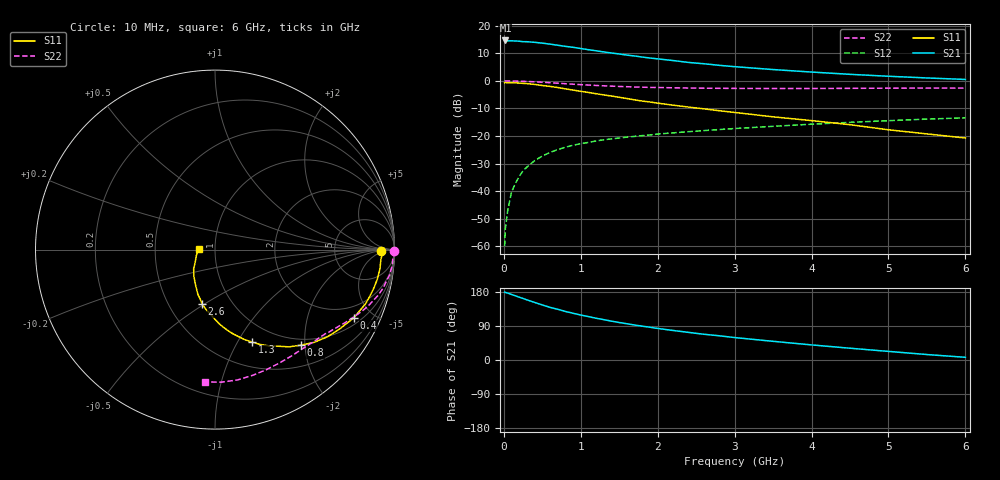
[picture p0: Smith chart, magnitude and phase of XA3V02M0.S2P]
! SIEMENS Discrete & RF Semiconductors
! BFY180
! Si NPN RF Bipolar Junction Transistor in MICRO-X
! VCE = 3 V  IC = 2 mA
! Common Emitter S-Parameters:  May  1997
# GHz  S  MA  R  50
!  f  S11  S21  S12  S22
! GHz  MAG  ANG  MAG  ANG  MAG  ANG  MAG  ANG
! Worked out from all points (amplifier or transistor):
!   36 points, 10 MHz to 6 GHz, reference 50 ohm
!   highest |S21| = 14.7 dB at 20 MHz (marker M1)
!   |S21| within 3 dB of that: start of sweep to 1.018 GHz
!   unconditionally stable (mu >= 1): 2.747 GHz to end of sweep
!   at 250 MHz: K = 0.12, MSG = 23.4 dB, |S12| = -32.6 dB
!   at 1.4 GHz: K = 0.69, MSG = 15.6 dB, |S12| = -21.1 dB
!   at 6 GHz: K = 1.07, MAG = 5.3 dB, |S12| = -13.4 dB
!   S11 on the Smith chart (normalised r, x): 10 MHz: 26, -2; 400 MHz: 1.31, -3.88; 800 MHz: 0.88, -1.91; 1.3 GHz: 0.77, -1.15; 2.6 GHz: 0.73, -0.49; 6 GHz: 0.83, +0.01
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0.01  0.9257 -0.4  5.296 179.1  0.001 82.6  0.9951 -0.3
0.02  0.9326 -1.3  5.411 178.3  0.0021 91.3  0.9958 -0.6
0.05  0.9261 -3.4  5.315 176.5  0.0044 84.4  0.9955 -1.6
0.1  0.9251 -6.7  5.321 173.0  0.0096 87.5  0.9913 -3.4
0.2  0.9109 -13.5  5.246 165.7  0.0184 81.5  0.9866 -6.6
0.25  0.9009 -16.8  5.145 162.4  0.0234 80.5  0.9827 -8.4
0.4  0.8616 -26.2  5.004 151.9  0.0356 73.7  0.9615 -12.8
0.5  0.8242 -32.3  4.837 145.3  0.0432 69.9  0.9443 -15.6
0.6  0.7935 -37.7  4.643 138.9  0.0502 67.1  0.9245 -18.1
0.8  0.7155 -48.1  4.225 128.1  0.0625 61.2  0.888 -22.7
0.9  0.6812 -52.7  4.066 123.3  0.0679 58.6  0.8699 -24.7
1.1  0.6165 -60.6  3.673 114.5  0.0764 55.1  0.839 -28.3
1.3  0.5553 -68.1  3.348 106.5  0.0853 51.5  0.8131 -31.5
1.5  0.5028 -74.8  3.071 98.9  0.0918 48.8  0.7918 -34.5
1.7  0.4517 -81.6  2.829 92.2  0.0983 47.1  0.7733 -37.3
2  0.394 -89.2  2.505 83.3  0.1084 44.5  0.7576 -41.3
2.2  0.3621 -93.9  2.339 77.9  0.1138 42.6  0.7487 -44.0
2.6  0.3106 -103.4  2.044 67.9  0.1251 39.9  0.7362 -49.0
3.5  0.2224 -119.4  1.604 49.3  0.1497 34.0  0.7266 -60.3
4.5  0.1601 -138.0  1.314 31.1  0.1767 26.8  0.7313 -73.4
5.5  0.109 -162.2  1.129 14.4  0.2023 19.2  0.7396 -87.4
6  0.0918 176.5  1.061 7.1  0.2135 15.0  0.7389 -94.4
